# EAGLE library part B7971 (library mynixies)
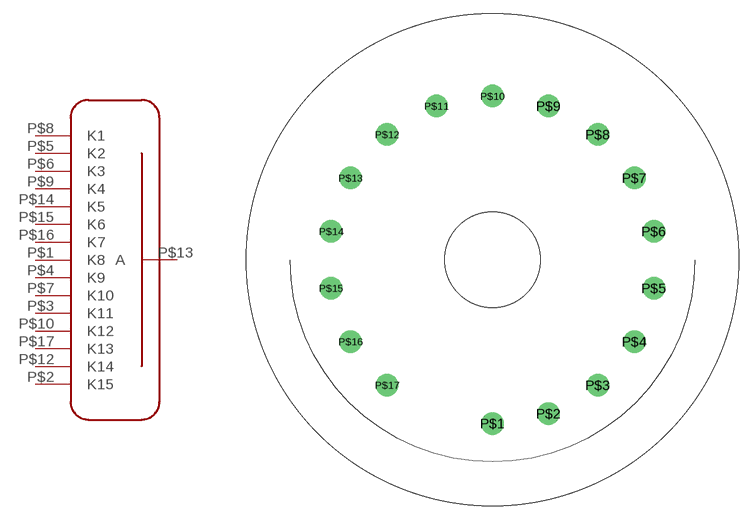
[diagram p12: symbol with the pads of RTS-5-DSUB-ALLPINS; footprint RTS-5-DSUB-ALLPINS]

Designator prefix NX

## B7971  [RTS-5-DSUB-ALLPINS]
P$1  K8  pas
P$2  K15  pas
P$3  K11  pas
P$4  K9  pas
P$5  K2  pas
P$6  K3  pas
P$7  K10  pas
P$8  K1  pas
P$9  K4  pas
P$10  K12  pas
P$12  K14  pas
P$13  A  pas
P$14  K5  pas
P$15  K6  pas
P$16  K7  pas
P$17  K13  pas

## Footprint RTS-5-DSUB-ALLPINS (pad centres in mm)
drill 1.6: P$1 0,-17.462; P$2 5.973,-16.409; P$3 11.225,-13.377; P$4 15.123,-8.731; P$5 17.197,-3.032; P$6 17.197,3.032; P$7 15.123,8.731; P$8 11.225,13.377; P$9 5.973,16.409; P$10 0,17.462; P$11 -5.973,16.409; P$12 -11.225,13.377; P$13 -15.123,8.731; P$14 -17.197,3.032; P$15 -17.197,-3.032; P$16 -15.123,-8.731; P$17 -11.225,-13.377
hole 10.16 at 0,0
